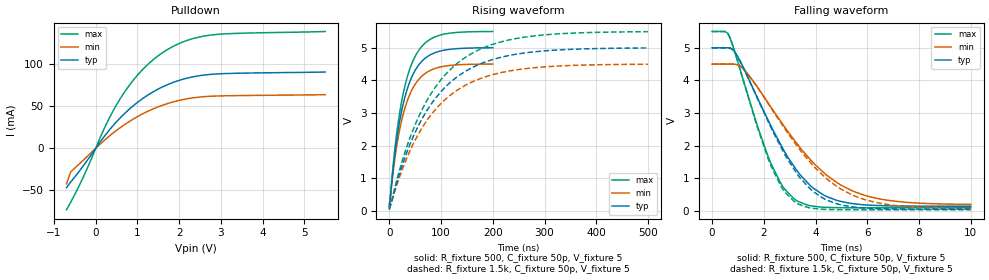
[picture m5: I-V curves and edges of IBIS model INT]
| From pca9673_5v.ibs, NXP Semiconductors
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[Model]   INT
Model_type Open_drain
Vref=5
Vmeas=2.5
Rref=1.6k
Cref=50p
C_comp   5.2p   5p   5.4p
[Temperature Range] 27   85   -40
[Voltage Range]   5   4.5   5.5
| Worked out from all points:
|   slope of the pulldown table from 0 to 0.75 V, typ, clamps not added: 17 ohm
|   falling waveform, R_fixture 500, C_fixture 50p, V_fixture 5: 20-80 % time 1.97ns typ, 2.6ns min, 1.39ns max; typ from 5 V to 0.139 V
|   falling waveform, R_fixture 1.5k, C_fixture 50p, V_fixture 5: 20-80 % time 1.94ns typ, 2.57ns min, 1.38ns max; typ from 5 V to 0.046 V
|   rising waveform, R_fixture 500, C_fixture 50p, V_fixture 5: 20-80 % time 35.1ns typ, 35.2ns min, 35.1ns max; typ from 0.139 V to 5 V
|   rising waveform, R_fixture 1.5k, C_fixture 50p, V_fixture 5: 20-80 % time 105ns typ, 105ns min, 105ns max; typ from 0.046 V to 4.99 V
[Pulldown]
-700mV    -46.85mA   -42.29mA   -73.04mA
-600mV    -40.09mA   -28.2mA    -64.29mA
-300mV    -21.02mA   -14.28mA   -34.53mA
200mV     13.79mA    9.177mA    23.06mA
400mV     26.03mA    17.52mA    42.92mA
600mV     36.84mA    25.02mA    59.95mA
800mV     46.31mA    31.73mA    74.52mA
1.1V      58.28mA    40.36mA    92.41mA
1.6V      73.01mA    51.21mA    113.7mA
2.1V      82.29mA    58.06mA    126.7mA
2.7V      87.7mA     61.77mA    134.3mA
5.5V      90.74mA    63.79mA    138.9mA
[Falling Waveform]
R_fixture=500
C_fixture=50p
V_fixture=5
V_fixture_min=4.5
V_fixture_max=5.5
0s        5V         4.5V       5.5V
606.1ps   5V         4.5V       5.447V
1.212ns   4.39V      4.353V     3.997V
2.222ns   2.689V     3.242V     1.547V
2.727ns   1.921V     2.659V     744.9mV
3.232ns   1.286V     2.111V     325mV
4.343ns   468.8mV    1.149V     106.1mV
5.556ns   207.4mV    568.6mV    91.02mV
7.071ns   147.1mV    291.7mV    90.25mV
10ns      138.8mV    194.8mV    90.23mV
[Falling Waveform]
R_fixture=1.5k
C_fixture=50p
V_fixture=5
V_fixture_min=4.5
V_fixture_max=5.5
0s        5V         4.5V       5.5V
505.1ps   5V         4.5V       5.498V
707.1ps   4.989V     4.5V       5.285V
1.212ns   4.386V     4.352V     3.984V
2.222ns   2.648V     3.222V     1.478V
2.727ns   1.853V     2.62V      662.2mV
3.232ns   1.195V     2.049V     246.4mV
4.343ns   360.9mV    1.042V     42.71mV
5.556ns   107.5mV    439.9mV    30.39mV
10ns      46.07mV    69.12mV    29.81mV
[Rising Waveform]
R_fixture=500
C_fixture=50p
V_fixture=5
V_fixture_min=4.5
V_fixture_max=5.5
0s        138.7mV    187.4mV    90.23mV
8.081ns   1.37V      1.261V     1.483V
12.12ns   1.904V     1.737V     2.075V
22.22ns   2.921V     2.643V     3.201V
28.28ns   3.363V     3.037V     3.691V
36.36ns   3.81V      3.436V     4.186V
52.53ns   4.372V     3.938V     4.807V
70.71ns   4.694V     4.226V     5.162V
96.97ns   4.891V     4.403V     5.381V
200ns     4.998V     4.498V     5.498V
[Rising Waveform]
R_fixture=1.5k
C_fixture=50p
V_fixture=5
V_fixture_min=4.5
V_fixture_max=5.5
0s        45.97mV    62.61mV    29.81mV
15.15ns   893.7mV    813.7mV    975.5mV
30.3ns    1.633V     1.477V     1.792V
60.61ns   2.739V     2.468V     3.012V
80.81ns   3.267V     2.942V     3.593V
101ns     3.671V     3.305V     4.039V
146.5ns   4.27V      3.842V     4.698V
197ns     4.624V     4.162V     5.088V
262.6ns   4.842V     4.357V     5.327V
500ns     4.993V     4.494V     5.492V
[Ramp]
R_load=1.6k
dV/dt_r   2.974E+0/1.675E-9   2.961E+0/1.840E-9   2.985E+0/1.482E-9
dV/dt_f   2.974E+0/8.642E-11   2.961E+0/1.513E-10   2.985E+0/1.040E-10
|[End   INT
